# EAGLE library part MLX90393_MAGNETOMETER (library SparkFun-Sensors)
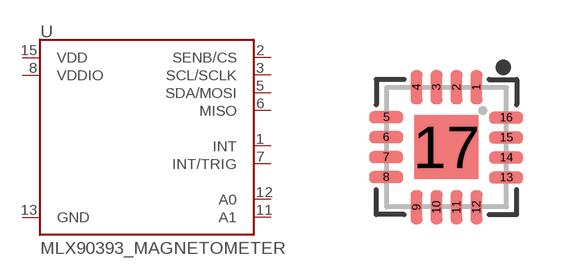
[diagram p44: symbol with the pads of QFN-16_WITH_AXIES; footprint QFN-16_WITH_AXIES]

Designator prefix -

## MLX90393_MAGNETOMETER (PROD_ID: SEN-13886)  [QFN-16_WITH_AXIES]
1  INT
2  SENB/CS
3  SCL/SCLK
5  SDA/MOSI
6  MISO
7  INT/TRIG
8  VDDIO
11  A1
12  A0
13  GND
15  VDD

## Footprint QFN-16_WITH_AXIES (pad centres in mm)
QFN-16 - 3.0mm x 3.0mm package for the MLX90393 Specifications: Pin count: 16 Pin pitch: .5mm Area: 3.0mm x 3.0mm Datasheet referenced for footprint
smd 0.3 x 0.85: 1 0.754,1.498; 2 0.254,1.498; 3 -0.246,1.498; 4 -0.746,1.498; 9 -0.746,-1.506; 10 -0.246,-1.506; 11 0.254,-1.506; 12 0.754,-1.506
smd 0.85 x 0.3: 5 -1.508,0.746; 6 -1.508,0.246; 7 -1.508,-0.254; 8 -1.508,-0.754; 13 1.496,-0.764; 14 1.496,-0.264; 15 1.496,0.236; 16 1.496,0.736
smd 1.6 x 1.6: 17 0,0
